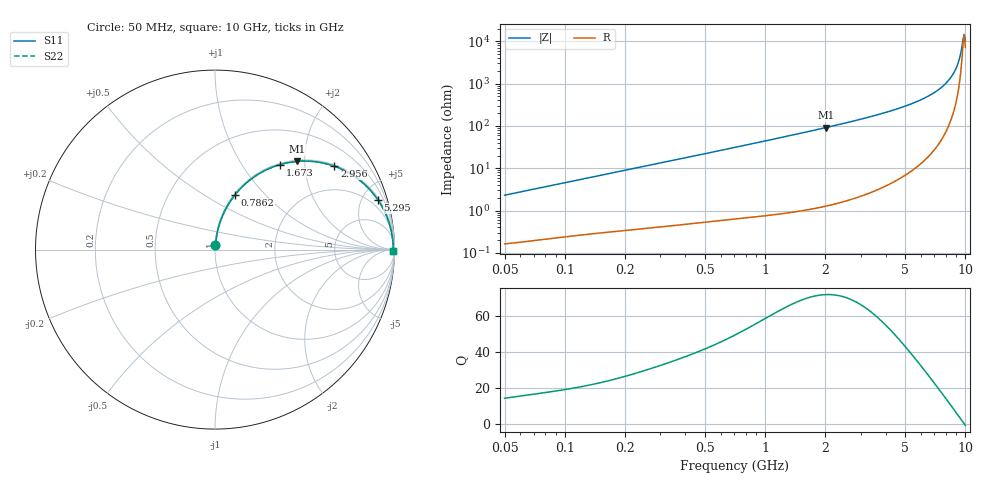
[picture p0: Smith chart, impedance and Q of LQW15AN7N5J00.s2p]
!Murata Part Number: LQW15AN7N5J00
!These Parameters are Measured in Series Mode Connection
!  o--[Z]--o
!Port1  Port2
!  o-------o
!Freq. Start=50[MHz] Stop=10[GHz], 401[Steps]
# Hz S RI R 50
!Freq.(Hz)	S 11(Real)	S 11(Imag)	S 21(Real)	S 21(Imag)	S 12(Real)	S 12(Imag)	S 22(Real)	S 22(Imag)
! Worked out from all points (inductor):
!   401 points, 50 MHz to 10 GHz, reference 50 ohm
!   read as one part in series: L = 7.3 nH near 51.34 MHz
!   highest Q = 71.9 at 2.013 GHz (marker M1), where L = 7.25 nH
!   self-resonance near 9.739 GHz
!   S11 on the Smith chart (normalised r, x): 50 MHz: 1.00, +0.05; 786.2 MHz: 1.01, +0.69; 1.673 GHz: 1.02, +1.50; 2.956 GHz: 1.04, +2.84; 5.295 GHz: 1.16, +6.49; 10 GHz: open
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5e7  0.00216 0.023  0.9978 -0.023  0.9978 -0.023  0.00216 0.023
1.214486e8  0.00563 0.0544  0.9944 -0.0544  0.9944 -0.0544  0.00563 0.0544
2.949953e8  0.0207 0.1278  0.9793 -0.1278  0.9793 -0.1278  0.0207 0.1278
7.071068e8  0.0935 0.2812  0.9065 -0.2812  0.9065 -0.2812  0.0935 0.2812
7.861503e8  0.1122 0.3061  0.8878 -0.3061  0.8878 -0.3061  0.1122 0.3061
1.154331e9  0.2116 0.4005  0.7884 -0.4005  0.7884 -0.4005  0.2116 0.4005
1.67264e9  0.3634 0.4739  0.6366 -0.4739  0.6366 -0.4739  0.3634 0.4739
1.717543e9  0.3763 0.4774  0.6237 -0.4774  0.6237 -0.4774  0.3763 0.4774
2.013439e9  0.4577 0.4913  0.5423 -0.4913  0.5423 -0.4913  0.4577 0.4913
2.956399e9  0.6655 0.4644  0.3345 -0.4644  0.3345 -0.4644  0.6655 0.4644
4.171863e9  0.8264 0.3694  0.1736 -0.3694  0.1736 -0.3694  0.8264 0.3694
5.295127e9  0.9077 0.2772  0.0923 -0.2772  0.0923 -0.2772  0.9077 0.2772
6.901252e9  0.9656 0.1621  0.0344 -0.1621  0.0344 -0.1621  0.9656 0.1621
7.571744e9  0.9782 0.1203  0.0218 -0.1203  0.0218 -0.1203  0.9782 0.1203
8.198065e9  0.9859 0.0841  0.0141 -0.0841  0.0141 -0.0841  0.9859 0.0841
8.644138e9  0.9895 0.0599  0.0105 -0.0599  0.0105 -0.0599  0.9895 0.0599
8.994549e9  0.9914 0.0417  0.00861 -0.0417  0.00861 -0.0417  0.9914 0.0417
9.236013e9  0.9923 0.0296  0.00771 -0.0296  0.00771 -0.0296  0.9923 0.0296
9.359165e9  0.9926 0.0235  0.00738 -0.0235  0.00738 -0.0235  0.9926 0.0235
9.610418e9  0.9931 0.0113  0.00693 -0.0113  0.00693 -0.0113  0.9931 0.0113
9.868415e9  0.9932 -0.000845  0.00678 0.000845  0.00678 0.000845  0.9932 -0.000845
1e10  0.9932 -0.00693  0.00682 0.00693  0.00682 0.00693  0.9932 -0.00693
